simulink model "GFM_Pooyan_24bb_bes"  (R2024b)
settings: Solver=FixedStepAuto  StartTime=0.0  StopTime=1  FixedStep=Ts  RelTol=1e-3
model workspace (MAT data in the model file):
  Po = 0
  b1 = 1000.38104695
  b2 = 1006.47399607
  b3 = 1006.95432939
  b4 = 996.322108769
  b5 = 995.669039411
  b6 = 1012.96535236
  b7 = 1007.5422409
  b8 = 993.960341463
  l1 = 8282.83466164
  l10 = 5511.54621883
  l11 = 8516.9845943
  l12 = 3533.51403234
  l13 = 1255.67117866
  l14 = 1105.23671469
  l15 = 955.492069576
  l16 = 1255.83166019
  l2 = 7767.51754481
  l3 = 6680.69860842
  l4 = 3013.93364227
  l5 = 912.604633733
  l6 = 706.803488619
  l7 = 1117.39027011
  l8 = 1674.30810947
  l9 = 1971.00014576
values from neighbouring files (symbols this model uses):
  alpha_p = 0.0005    [initialcondition_gfm_Pooyan.m]    (also in initialcondition_Pooyan.m = 0.0001)
  alpha_q = 0.0001    [initialcondition_gfm_Pooyan.m]    (also in initialcondition_Pooyan.m)
  Cf = 50e-6    (= 5e-05)    [initialcondition_gfm_Pooyan.m]    (also in initialcondition_Pooyan.m)
  I_instant_limit_peak = I_instant_limit_rms * sqrt(2)    [initialcondition_gfm_Pooyan.m]
  I_overload_limit = 1.2 * I_rated_rms    [initialcondition_gfm_Pooyan.m]
  Kicc = 314.159    [initialcondition_gfm_Pooyan.m]    (also in initialcondition_Pooyan.m)
  Kivc = 400    [initialcondition_gfm_Pooyan.m]    (also in initialcondition_Pooyan.m)
  Kpcc = 31.4159    [initialcondition_gfm_Pooyan.m]    (also in initialcondition_Pooyan.m)
  Kpvc = 0.5    [initialcondition_gfm_Pooyan.m]    (also in initialcondition_Pooyan.m)
  Lf = 10e-3    (= 0.01)    [initialcondition_gfm_Pooyan.m]    (also in initialcondition_Pooyan.m)
  Lg = X_BY_R*Rg/(wn)    [initialcondition_gfm_Pooyan.m]    (also in DER_param.m = (X_BY_R_gfl * Rg) / wn_gfl; initialcondition_Pooyan.m)
  Pn = 20000    [initialcondition_gfm_Pooyan.m]    (also in initialcondition_Pooyan.m)
  Qn = 0    [initialcondition_gfm_Pooyan.m]    (also in initialcondition_Pooyan.m)
  R = (3*Vg^2)/(2*Pn)    (= 8.000067)    [initialcondition_gfm_Pooyan.m]    (also in MC2.m = (8760*SS-sum(Tdown))/(8760*SS); initialcondition_Pooyan.m)
  R_extra = (3*Vg^2)/(2*P_extra)    (= 10.666756)    [initialcondition_gfm_Pooyan.m]
  Rf = 0.1    [initialcondition_gfm_Pooyan.m]    (also in initialcondition_Pooyan.m)
  Rg = (3*Vg^2)/(2*SCR*sqrt(1+X_BY_R^2)*Pn)    [initialcondition_gfm_Pooyan.m]    (also in DER_param.m = (3 * Vg_gfl^2) / (2 * SCR_gfl * sqrt(1 + X_BY_R_gfl^2) * Pn_; initialcondition_Pooyan.m)
  tau_p = 0.031415    [initialcondition_gfm_Pooyan.m]    (also in initialcondition_Pooyan.m)
  tau_q = 0.031415    [initialcondition_gfm_Pooyan.m]    (also in initialcondition_Pooyan.m)
  Ts = 50e-6    (= 5e-05)    [initialcondition_gfm_Pooyan.m]    (also in initialcondition_Pooyan.m)
  Vdc = 700    [initialcondition_gfm_Pooyan.m]    (also in initialcondition_Pooyan.m)
  Vg = 326.6    [initialcondition_gfm_Pooyan.m]    (also in initialcondition_Pooyan.m)
  wn = 2*pi*50    (= 314.159265359)    [initialcondition_gfm_Pooyan.m]    (also in initialcondition_Pooyan.m)
undefined symbols (not defined in the file or in its folder): Ion, Lithium
libraries: simulink x6, slpidlib x5, spsThreePhaseBreakerLib x3, spsabctodq0Lib x3, spsGroundLib x3, spsThreePhaseSeriesRLCBranchLib x3, spsThreePhaseVIMeasurementLib x3, spsIGBTDiodeLib x2, spsSeriesRLCBranchLib x2, spsThreePhaseParallelRLCBranchLib x2, spsThreePhaseSourceLib x1, spsBatteryLib x1
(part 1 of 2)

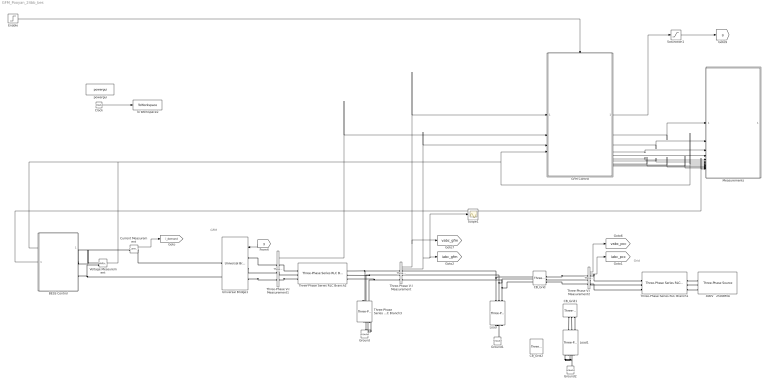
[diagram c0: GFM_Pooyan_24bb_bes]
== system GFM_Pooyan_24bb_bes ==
  note: Grid
  note: GFM
  400V   2500MVA : spsThreePhaseSourceLib/Three-Phase Source  InternalConnection=Yg  VoltagePhases=off  Voltage=Vg*sqrt(3/2)  PhaseAngle=0  Voltage_phases=[25e3 25e3 25e3]/sqrt(3)  PhaseAngles_phases=[0 -120 +120]  Frequency=50  NonIdealSource=on  SpecifyImpedance=off  Resistance=0  Inductance=0  ShortCircuitLevel=2500e6  BaseVoltage=Vg*sqrt(3/2)  XRratio=7  BusType=swing  Pref=0  Qref=0  Prefabc=[10e3, 10e3, 10e3]  Qrefabc=[0, 0, 0]  Qmin=-inf  Qmax=inf
  BESS Control : Subsystem
  CB_Grid : spsThreePhaseBreakerLib/Three-Phase Breaker  InitialState=open  SwitchA=on  SwitchB=on  SwitchC=on  SwitchTimes=[0.5]  External=off  BreakerResistance=0.01  SnubberResistance=1e6  SnubberCapacitance=inf  Measurements=None
  CB_Grid1 : spsThreePhaseBreakerLib/Three-Phase Breaker  Commented=on  InitialState=open  SwitchA=on  SwitchB=on  SwitchC=on  SwitchTimes=[1.5]  External=off  BreakerResistance=0.01  SnubberResistance=1e6  SnubberCapacitance=inf  Measurements=None
  CB_Grid2 : spsThreePhaseBreakerLib/Three-Phase Breaker  Commented=on  InitialState=closed  SwitchA=on  SwitchB=on  SwitchC=on  SwitchTimes=[1]  External=on  BreakerResistance=0.01  SnubberResistance=1e6  SnubberCapacitance=inf  Measurements=None
  Clock : Clock
  Current Measurement : spsCurrentMeasurementLib/Current Measurement  PhasorSimulation=off  OutputType=Complex  PSBequivalent=0
  Enable : Step  Time=0  SampleTime=0
  GFM Control : Subsystem
  Ground : spsGroundLib/Ground  LConnTagsString=a
  Ground1 : spsGroundLib/Ground  LConnTagsString=a
  Ground2 : spsGroundLib/Ground  Commented=on  LConnTagsString=a
  Load : spsThreePhaseParallelRLCBranchLib/Three-Phase Parallel RLC Branch  LConnTagsString=A|B|C  RConnTagsString=A|B|C  BranchType=R  Resistance=R  Inductance=1e-3  Capacitance=1e-6  Measurements=None
  Load1 : spsThreePhaseParallelRLCBranchLib/Three-Phase Parallel RLC Branch  Commented=on  LConnTagsString=A|B|C  RConnTagsString=A|B|C  BranchType=R  Resistance=R_extra  Inductance=1e-3  Capacitance=1e-6  Measurements=None
  Measurements : Subsystem
  Saturation1 : Saturate  UpperLimit=1  LowerLimit=-1
  Scope1 : Scope
  Three-Phase Series RLC Branch1 : spsThreePhaseSeriesRLCBranchLib/Three-Phase Series RLC Branch  LConnTagsString=A|B|C  RConnTagsString=A|B|C  BranchType=RL  Resistance=Rg  Inductance=Lg  Capacitance=1e-6  Measurements=None
  Three-Phase Series RLC Branch2 : spsThreePhaseSeriesRLCBranchLib/Three-Phase Series RLC Branch  LConnTagsString=A|B|C  RConnTagsString=A|B|C  BranchType=RL  Resistance=Rf  Inductance=Lf  Capacitance=1e-6  Measurements=None
  Three-Phase Series RLC Branch3 : spsThreePhaseSeriesRLCBranchLib/Three-Phase Series RLC Branch  LConnTagsString=A|B|C  RConnTagsString=A|B|C  BranchType=C  Resistance=0.1  Inductance=280e-3  Capacitance=Cf  Measurements=None
  Three-Phase V-I Measurement : spsThreePhaseVIMeasurementLib/Three-Phase V-I Measurement  VoltageMeasurement=phase-to-ground  SetLabelV=off  LabelV=Vabc  Vpu=off  VpuLL=off  CurrentMeasurement=yes  SetLabelI=off  LabelI=Iabc  Ipu=off  Pbase=100e6  Vbase=500e3  OutputType=Complex  PhasorSimulation=off  PSBequivalent=0
  Three-Phase V-I Measurement1 : spsThreePhaseVIMeasurementLib/Three-Phase V-I Measurement  VoltageMeasurement=no  SetLabelV=off  LabelV=Vabc  Vpu=off  VpuLL=off  CurrentMeasurement=yes  SetLabelI=off  LabelI=Iabc  Ipu=off  Pbase=100e6  Vbase=500e3  OutputType=Complex  PhasorSimulation=off  PSBequivalent=0
  Three-Phase V-I Measurement2 : spsThreePhaseVIMeasurementLib/Three-Phase V-I Measurement  VoltageMeasurement=phase-to-ground  SetLabelV=off  LabelV=Vabc  Vpu=off  VpuLL=off  CurrentMeasurement=yes  SetLabelI=off  LabelI=Iabc  Ipu=off  Pbase=100e6  Vbase=500e3  OutputType=Complex  PhasorSimulation=off  PSBequivalent=0
  To Workspace2 : ToWorkspace  VariableName=t  SampleTime=-1
  Universal Bridge1 : spsUniversalBridgeLib/Universal Bridge  Arms=3  SnubberResistance=1e5  SnubberCapacitance=inf  Device=Average-model based VSC  Ron=1e-3  Lon=0  ForwardVoltages="[  0  0  ]"  ForwardVoltage=0  GTOparameters=[ 10e-6 , 20e-6 ]  IGBTparameters=[ 1e-6 , 2e-6 ]  Measurements=None  Measurements_2=None  converterType=Rectifier
  Voltage Measurement : spsVoltageMeasurementLib/Voltage Measurement  PhasorSimulation=off  OutputType=Complex  PSBequivalent=0
  powergui : spspowerguiLib/powergui  Priority=1  SimulationMode=Discrete  SampleTime=Ts  frequency=50  Iterations=50  frequencyindice=0  Pbase=100e6  ErrMax=1e-4  UnitsV=kV  UnitsW=MW  buscounter=0  FunctionMessages=off  echomessages=off  EnableUseOfTLC=off  CurrentSourceSwitches=off  DisableSnubberDevices=off  DisableRonSwitches=off  DisableVfSwitches=off  DisplayEquations=off  AutomaticDiscreteSolvers=off  SolverType=Tustin  Interpol=off  ExternalGateDelay=off  methode=off  Ts=0  x0status=blocks  SPID=off  SwTol=0  HookPort=off  NonlinearTolerance=0  nMaxIteration=15  ContinueOnMaxIteration=off  RestoreLinks=warning  ResistiveCurrentMeasurement=off  Frange=[0:2:500]  Ylog=off  Xlog=on  ShowGrid=off  save=off  variable=ZData  structure=0  ZoomFFT=on  StartTime=0.0  cycles=1  DisplayStyle=1  fundamental=60  FreqAxis=off  MaxFrequency=1000  frequencyindicesteady=1  RmsSteady=1  display=off
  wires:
  [g] -> Universal Bridge1/1
  Clock/1 -> To Workspace2/1
  Three-Phase V-I Measurement2/1 -> [vabc_pcc]
  Current Measurement/1 -> [i_demand]
  Three-Phase V-I Measurement/1 -> [vabc_gfm], GFM Control/1(v_abc_gfm)
  Three-Phase V-I Measurement/2 -> Scope1/1, [iabc_gfm], GFM Control/3(i_abc_gfm)
  Three-Phase V-I Measurement1/1 -> GFM Control/2(i_abc_filter)
  Enable/1 -> GFM Control/Enable
  Voltage Measurement/1 -> Measurements/7(In7), GFM Control/4(vdc), BESS Control/1(vbus)
  GFM Control/1(g) -> Saturation1/1
  GFM Control/2(Outport) -> Measurements/1(In1)
  GFM Control/3(Outport1) -> Measurements/2(In2)
  GFM Control/4(Outport2) -> Measurements/3(In3)
  GFM Control/5(Outport3) -> Measurements/4(In4)
  GFM Control/6(Outport4) -> Measurements/5(In5)
  GFM Control/7(Outport5) -> Measurements/6(In6)
  Three-Phase V-I Measurement2/2 -> [iabc_pcc]
  GFM Control/9(CB) -> Measurements/8(CB)
  GFM Control/10(peak) -> Measurements/9(peak)
  GFM Control/11(rms) -> Measurements/10(rms)
  BESS Control/1(I_ref) -> Measurements/11(I_ref)
  Saturation1/1 -> [g]
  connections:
  Three-Phase V-I Measurement/LConn3 -- Three-Phase Series RLC Branch3/LConn3 -- Three-Phase Series RLC Branch2/RConn3
  Three-Phase V-I Measurement/LConn1 -- Three-Phase Series RLC Branch2/RConn1 -- Three-Phase Series RLC Branch3/LConn1
  Ground/LConn1 -- Three-Phase Series RLC Branch3/RConn1 -- Three-Phase Series RLC Branch3/RConn2 -- Three-Phase Series RLC Branch3/RConn3
  Three-Phase V-I Measurement1/RConn1 -- Three-Phase Series RLC Branch2/LConn1
  Three-Phase V-I Measurement1/RConn2 -- Three-Phase Series RLC Branch2/LConn2
  Three-Phase V-I Measurement/LConn2 -- Three-Phase Series RLC Branch3/LConn2 -- Three-Phase Series RLC Branch2/RConn2
  Three-Phase V-I Measurement1/RConn3 -- Three-Phase Series RLC Branch2/LConn3
  Load/LConn1 -- Three-Phase V-I Measurement/RConn1 -- CB_Grid/LConn1
  Load/LConn2 -- CB_Grid/LConn2 -- Three-Phase V-I Measurement/RConn2
  Load/LConn3 -- CB_Grid/LConn3 -- Three-Phase V-I Measurement/RConn3
  Three-Phase Series RLC Branch1/RConn1 -- 400V   2500MVA/RConn1
  Three-Phase Series RLC Branch1/RConn2 -- 400V   2500MVA/RConn2
  Three-Phase Series RLC Branch1/RConn3 -- 400V   2500MVA/RConn3
  Three-Phase V-I Measurement2/RConn1 -- Three-Phase Series RLC Branch1/LConn1
  Three-Phase V-I Measurement2/RConn2 -- Three-Phase Series RLC Branch1/LConn2
  Three-Phase V-I Measurement2/RConn3 -- Three-Phase Series RLC Branch1/LConn3
  CB_Grid/RConn1 -- Three-Phase V-I Measurement2/LConn1
  CB_Grid/RConn2 -- Three-Phase V-I Measurement2/LConn2
  CB_Grid/RConn3 -- Three-Phase V-I Measurement2/LConn3
  Load/RConn3 -- Ground1/LConn1 -- Load/RConn2 -- Load/RConn1
  Universal Bridge1/LConn1 -- Three-Phase V-I Measurement1/LConn1
  Universal Bridge1/LConn2 -- Three-Phase V-I Measurement1/LConn2
  Universal Bridge1/LConn3 -- Three-Phase V-I Measurement1/LConn3
  Voltage Measurement/LConn2 -- Universal Bridge1/RConn2 -- BESS Control/LConn2
  BESS Control/LConn1 -- Current Measurement/LConn1 -- Voltage Measurement/LConn1
  Current Measurement/RConn1 -- Universal Bridge1/RConn1
  Load1/RConn1 -- Load1/RConn3 -- Ground2/LConn1 -- Load1/RConn2
  Load1/LConn1 -- CB_Grid1/LConn1
  Load1/LConn2 -- CB_Grid1/LConn2
  Load1/LConn3 -- CB_Grid1/LConn3

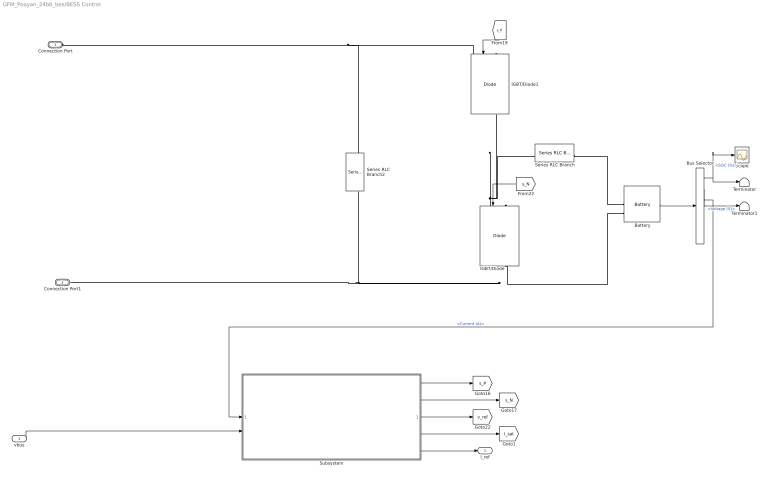
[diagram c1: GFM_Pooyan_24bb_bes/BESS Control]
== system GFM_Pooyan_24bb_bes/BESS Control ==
  vbus : Inport
  Battery : spsBatteryLib/Battery  BatType=Lithium-Ion  NomV=385  NomQ=52  SOC=90  Batt_Tr=1  PresetModel=on  MaxQ=52  MinV=288.75  FullV=448.135  Dis_rate=22.6087  R=0.074038  Normal_OP=47.0261  expZone="[415.9486      2.554783]"
  Bus Selector : BusSelector  OutputSignals=SOC (%),Voltage (V),Current (A)
  IGBT/Diode : spsIGBTDiodeLib/IGBT//Diode  Ron=1e-3  Rs=1e5  Cs=inf  Measurements=off
  IGBT/Diode1 : spsIGBTDiodeLib/IGBT//Diode  Ron=1e-3  Rs=1e5  Cs=inf  Measurements=off
  Scope : Scope
  Series RLC Branch : spsSeriesRLCBranchLib/Series RLC Branch  LConnTagsString=__new0  RConnTagsString=__new0  BranchType=RL  Resistance=0.02  Inductance=1.8e-3  SetiL0=off  InitialCurrent=0  Capacitance=1e-6  Setx0=off  InitialVoltage=0  Measurements=None
  Series RLC Branch2 : spsSeriesRLCBranchLib/Series RLC Branch  LConnTagsString=__new0  RConnTagsString=__new0  BranchType=RC  Resistance=0.05  Inductance=1e-3  SetiL0=off  InitialCurrent=0  Capacitance=470e-6  Setx0=on  InitialVoltage=385  Measurements=None
  Subsystem : Subsystem
  Terminator : Terminator
  Terminator1 : Terminator
  Connection Port : PMIOPort  Side=Left
  Connection Port1 : PMIOPort  Port=2  Side=Left
  I_ref : Outport
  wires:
  [s_N] -> IGBT/Diode/1
  Battery/1 -> Bus Selector/1
  [s_P] -> IGBT/Diode1/1
  Bus Selector/3 -> Subsystem/1(i_bat)  "<Current (A)>"
  Bus Selector/1 -> Scope/1, Terminator/1  "<SOC (%)>"
  Bus Selector/2 -> Terminator1/1  "<Voltage (V)>"
  Subsystem/1(P) -> [s_P]
  Subsystem/2(Out2) -> [s_N]
  Subsystem/3(Out3) -> [v_ref]
  vbus/1 -> Subsystem/2(Inport)
  Subsystem/4(MAX_CURRENT) -> [I_sat]
  Subsystem/5(I_ref) -> I_ref/1
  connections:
  IGBT/Diode/LConn1 -- Series RLC Branch/LConn1 -- IGBT/Diode1/RConn1
  Battery/LConn2 -- Series RLC Branch2/RConn1 -- Connection Port1/RConn1 -- IGBT/Diode/RConn1
  Connection Port/RConn1 -- Series RLC Branch2/LConn1 -- IGBT/Diode1/LConn1
  Battery/LConn1 -- Series RLC Branch/RConn1

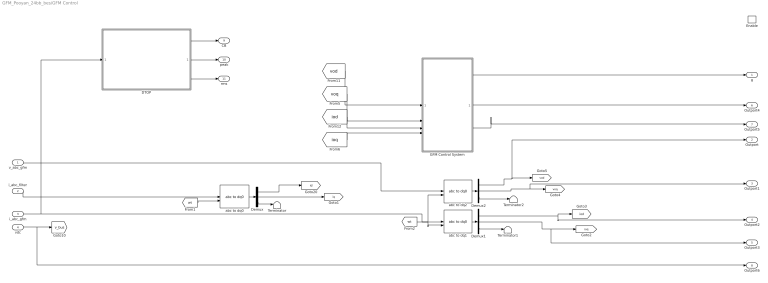
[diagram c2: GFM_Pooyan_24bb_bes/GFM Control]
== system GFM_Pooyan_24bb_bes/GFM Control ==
  v_abc_gfm : Inport
  i_abc_filter : Inport  Port=2
  i_abc_gfm : Inport  Port=3
  vdc : Inport  Port=4
  Enable : EnablePort  StatesWhenEnabling=reset
  DTOP : Subsystem
  Demux : Demux  Outputs=3
  Demux1 : Demux  Outputs=3
  Demux2 : Demux  Outputs=3
  GFM Control System : Subsystem
  Terminator : Terminator
  Terminator1 : Terminator
  Terminator2 : Terminator
  abc to dq0 : spsabctodq0Lib/abc to dq0  Alignment=90 degrees behind phase A axis
  abc to dq1 : spsabctodq0Lib/abc to dq0  Alignment=90 degrees behind phase A axis
  abc to dq2 : spsabctodq0Lib/abc to dq0  Alignment=90 degrees behind phase A axis
  g : Outport
  Outport : Outport  Port=2
  Outport1 : Outport  Port=3
  Outport2 : Outport  Port=4
  Outport3 : Outport  Port=5
  Outport4 : Outport  Port=6
  Outport5 : Outport  Port=7
  Outport6 : Outport  Port=8
  CB : Outport  Port=9
  peak : Outport  Port=10
  rms : Outport  Port=11
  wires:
  Demux1/2 -> Outport3/1, [ioq]
  [vod] -> GFM Control System/1(vod)
  Demux1/1 -> Outport2/1, [iod]
  Demux2/3 -> Terminator2/1
  Demux2/1 -> Outport/1, [vod]
  abc to dq2/1 -> Demux2/1
  Demux/1 -> [id]
  Demux/2 -> [iq]
  Demux2/2 -> Outport1/1, [voq]
  [ioq] -> GFM Control System/4(ioq)
  [wt] -> abc to dq2/2, abc to dq1/2
  i_abc_filter/1 -> abc to dq0/1
  [voq] -> GFM Control System/2(voq)
  [iod] -> GFM Control System/3(iod)
  abc to dq1/1 -> Demux1/1
  Demux/3 -> Terminator/1
  abc to dq0/1 -> Demux/1
  Demux1/3 -> Terminator1/1
  GFM Control System/1(g) -> g/1
  i_abc_gfm/1 -> DTOP/1(In), abc to dq1/1
  v_abc_gfm/1 -> abc to dq2/1
  vdc/1 -> Outport6/1, [v_bus]
  GFM Control System/3(Outport1) -> Outport5/1
  GFM Control System/2(Outport) -> Outport4/1
  [wt] -> abc to dq0/2
  DTOP/1(CB) -> CB/1
  DTOP/3(rms) -> rms/1
  DTOP/2(peak) -> peak/1

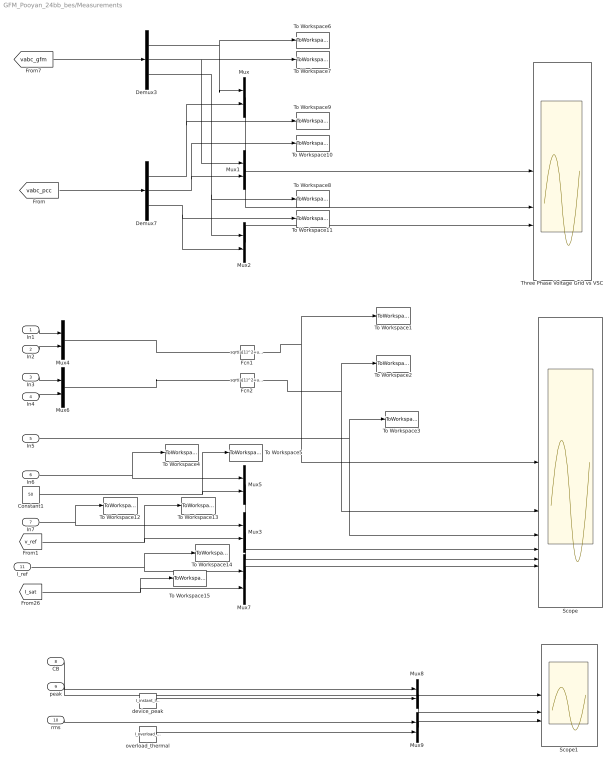
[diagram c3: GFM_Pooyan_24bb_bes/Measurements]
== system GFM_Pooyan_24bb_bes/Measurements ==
  In1 : Inport
  In2 : Inport  Port=2
  In3 : Inport  Port=3
  In4 : Inport  Port=4
  In5 : Inport  Port=5
  In6 : Inport  Port=6
  In7 : Inport  Port=7
  CB : Inport  Port=8
  peak : Inport  Port=9
  rms : Inport  Port=10
  I_ref : Inport  Port=11
  Constant1 : Constant  Value=50
  Demux3 : Demux  Outputs=3
  Demux7 : Demux  Outputs=3
  Fcn1 : Fcn  Expr=sqrt(u[1]^2+u[2]^2)
  Fcn2 : Fcn  Expr=sqrt(u[1]^2+u[2]^2)
  Mux{,1..9} (10 alike) : Mux  Inputs=2
  Scope : Scope  NumInputPorts=6
  Scope1 : Scope  NumInputPorts=3
  Three Phase Voltage Grid vs VSC : Scope  NumInputPorts=3
  To Workspace1 : ToWorkspace  VariableName=vo_GFM  SaveFormat=Timeseries  SampleTime=-1
  To Workspace10 : ToWorkspace  VariableName=Vb_grid  SaveFormat=Timeseries  SampleTime=-1
  To Workspace11 : ToWorkspace  VariableName=Vc_grid  SaveFormat=Timeseries  SampleTime=-1
  To Workspace12 : ToWorkspace  VariableName=vdc_meas_bess  SaveFormat=Timeseries  SampleTime=-1
  To Workspace13 : ToWorkspace  VariableName=vdc_set_bess  SaveFormat=Timeseries  SampleTime=-1
  To Workspace14 : ToWorkspace  VariableName=iref_bess  SaveFormat=Timeseries  SampleTime=-1
  To Workspace15 : ToWorkspace  VariableName=isat_bess  SaveFormat=Timeseries  SampleTime=-1
  To Workspace2 : ToWorkspace  VariableName=io_GFM  SaveFormat=Timeseries  SampleTime=-1
  To Workspace3 : ToWorkspace  VariableName=po_GFM1  SaveFormat=Timeseries  SampleTime=-1
  To Workspace4 : ToWorkspace  VariableName=fmeas_GFM  SaveFormat=Timeseries  SampleTime=-1
  To Workspace5 : ToWorkspace  VariableName=fset_GFM  SaveFormat=Timeseries  SampleTime=-1
  To Workspace6 : ToWorkspace  VariableName=Va_gfm  SaveFormat=Timeseries  SampleTime=-1
  To Workspace7 : ToWorkspace  VariableName=Vb_gfm  SaveFormat=Timeseries  SampleTime=-1
  To Workspace8 : ToWorkspace  VariableName=Vc_gfm  SaveFormat=Timeseries  SampleTime=-1
  To Workspace9 : ToWorkspace  VariableName=Va_grid  SaveFormat=Timeseries  SampleTime=-1
  device_peak : Constant  Value=I_instant_limit_peak
  overload_thermal : Constant  Value=I_overload_limit
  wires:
  [vabc_gfm] -> Demux3/1
  Constant1/1 -> To Workspace5/1, Mux5/2
  [vabc_pcc] -> Demux7/1
  Demux3/2 -> To Workspace7/1, Mux1/1
  In1/1 -> Mux4/1
  In2/1 -> Mux4/2
  Demux3/1 -> To Workspace6/1, Mux/1
  In3/1 -> Mux6/1
  In4/1 -> Mux6/2
  Mux4/1 -> Fcn1/1
  Demux3/3 -> Mux2/1, To Workspace8/1
  Demux7/1 -> Mux/2, To Workspace9/1
  Demux7/2 -> To Workspace10/1, Mux1/2
  [v_ref] -> To Workspace13/1, Mux3/2
  Demux7/3 -> Mux2/2, To Workspace11/1
  Mux6/1 -> Fcn2/1
  In6/1 -> To Workspace4/1, Mux5/1
  In7/1 -> To Workspace12/1, Mux3/1
  [I_sat] -> To Workspace15/1, Mux7/2
  Mux/1 -> Three Phase Voltage Grid vs VSC/1
  Mux1/1 -> Three Phase Voltage Grid vs VSC/2
  Mux2/1 -> Three Phase Voltage Grid vs VSC/3
  Fcn1/1 -> To Workspace1/1, Scope/1
  Fcn2/1 -> To Workspace2/1, Scope/2
  In5/1 -> To Workspace3/1, Scope/3
  Mux5/1 -> Scope/4
  Mux7/1 -> Scope/6
  Mux3/1 -> Scope/5
  CB/1 -> Scope1/1
  peak/1 -> Mux8/1
  device_peak/1 -> Mux8/2
  Mux8/1 -> Scope1/2
  rms/1 -> Mux9/1
  overload_thermal/1 -> Mux9/2
  Mux9/1 -> Scope1/3
  I_ref/1 -> To Workspace14/1, Mux7/1

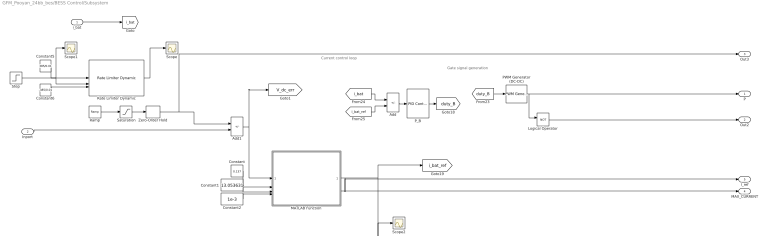
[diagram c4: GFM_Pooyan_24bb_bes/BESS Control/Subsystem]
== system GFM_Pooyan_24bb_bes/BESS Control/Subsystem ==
  note: Current control loop
  note: Gate signal generation
  i_bat : Inport
  Inport : Inport  Port=2
  Add : Sum  Inputs=+-
  Add1 : Sum  Inputs=+-
  Constant : Constant  Value=0.137
  Constant1 : Constant  Value=13.053631
  Constant2 : Constant  Value=1e-3
  Constant5 : Constant  Commented=on  Value=385/0.01
  Constant6 : Constant  Commented=on  Value=-385/0.01
  Logical Operator : Logic  Operator=NOT  AllPortsSameDT=off  OutDataTypeStr=boolean
  MATLAB Function : MATLAB Function  TreatAsAtomicUnit=on
  PWM Generator (DC-DC) : spsPWMGeneratorDCDCLib/PWM Generator (DC-DC)  Fsw=10000  Ts=1/10000
  P_B : slpidlib/PID Controller  Controller=PI  Form=Parallel  TimeDomain=Discrete-time  UseExternalTs=off  SampleTime=200e-6  IntegratorMethod=Forward Euler  FilterMethod=Forward Euler  ControllerParametersSource=internal  P=0.015756  I=0.179520  UseKiTs=off  D=0  UseExternalDerivativeSource=off  N=100  UseFilter=on  TunerSelectOption=Transfer Function Based (PID Tuner App)  InitialConditionSource=internal  InitialConditionForIntegrator=0  InitialConditionForFilter=0  DifferentiatorICPrevScaledInput=0  ExternalReset=none  TrackingMode=off  Kt=1  LimitOutput=on  SatLimitsSource=internal  UpperSaturationLimit=0.95  LowerSaturationLimit=0  LinearizeAsGain=off  AntiWindupMode=none  Kb=1  LimitIntegrator=off  UpperIntegratorSaturationLimit=inf  LowerIntegratorSaturationLimit=-inf  POutMin=[]  POutMax=[]  IOutMin=[]  IOutMax=[]  DOutMin=[]  DOutMax=[]  NOutMin=[]  NOutMax=[]  SumOutMin=[]  SumOutMax=[]  SaturationOutMin=[]  SaturationOutMax=[]  PParamMin=[]  PParamMax=[]  IParamMin=[]  IParamMax=[]  DParamMin=[]  DParamMax=[]  NParamMin=[]  NParamMax=[]  KbParamMin=[]  KbParamMax=[]  KtParamMin=[]  KtParamMax=[]  KbOutMin=[]  KbOutMax=[]  KtOutMin=[]  KtOutMax=[]  IntegratorOutMin=[]  IntegratorOutMax=[]  FilterOutMin=[]  FilterOutMax=[]  SumI1OutMin=[]  SumI1OutMax=[]  SumI2OutMin=[]  SumI2OutMax=[]  SumI3OutMin=[]  SumI3OutMax=[]  SumI4OutMin=[]  SumI4OutMax=[]  SumDOutMin=[]  SumDOutMax=[]  DifferentiatorOutMin=[]  DifferentiatorOutMax=[]  FilterDiffOutCoefMin=[]  FilterDiffOutCoefMax=[]  ReciprocalOutMin=[]  ReciprocalOutMax=[]  SumDenOutMin=[]  SumDenOutMax=[]  SumNumOutMin=[]  SumNumOutMax=[]  DivideOutMin=[]  DivideOutMax=[]  UdiffTsProdOutMin=[]  UdiffTsProdOutMax=[]  NTsProdOutMin=[]  NTsProdOutMax=[]  UintegralTsProdOutMin=[]  UintegralTsProdOutMax=[]  UngainTsProdOutMin=[]  UngainTsProdOutMax=[]  ClampingZeroOutDataTypeStr=Inherit: Inherit via back propagation  ClampingZeroOutMin=[]  ClampingZeroOutMax=[]  FilterDenConstantOutDataTypeStr=Inherit: Inherit via back propagation  FilterDenConstantOutMin=[]  FilterDenConstantOutMax=[]  PCopyOutDataTypeStr=Inherit: Inherit via back propagation  PCopyOutMin=[]  PCopyOutMax=[]  NCopyOutDataTypeStr=Inherit: Inherit via back propagation  NCopyOutMin=[]  NCopyOutMax=[]  IntegratorContinuousStateAttributes=''  IntegratorStateMustResolveToSignalObject=off  IntegratorRTWStateStorageClass=Auto  FilterContinuousStateAttributes=''  FilterStateMustResolveToSignalObject=off  FilterRTWStateStorageClass=Auto  ParallelPVariant=InternalParameters  IdealPVariant=Disabled  IVariant=InternalParameters  DVariant=Disabled  IntegratorVariant=Discrete  SatVariant=Enabled  AWVariant=Passthrough  PCopyVariant=Disabled  TRVariant=Disabled  FdbkBlocksVariant=Forward  IdealPFdbkVariant=Disabled  SatFdbkVariant=Disabled  DerivativeFilterVariant=Disabled  NVariant=Disabled  NCopyVariant=Disabled_SignalSpec  FilterICVariant=Disabled  IntegratorICVariant=InternalICs  ExternalResetVariant=Disabled  TRSumVariant=Passthrough  SumFdbkVariant=Disabled  SumVariant=Sum_PI  TsampFilterVariant=InternalTs  TsampNgainVariant=Passthrough  TsampIntegralVariant=Disabled_SignalSpec  ExternalSaturationOutDataTypeStr=Inherit: Same as second input  DerivativeSourceVariant=Disabled  PreIntVariant=InternalPreInt
  Ramp : simulink/Sources/Ramp  slope=315/0.01  start=0  InitialOutput=385
  Rate Limiter Dynamic : simulink/Discontinuities/Rate Limiter Dynamic  Commented=on
  Saturation : Saturate  UpperLimit=700  LowerLimit=-385
  Scope : Scope
  Scope1 : Scope
  Scope2 : Scope
  Step : Step  Commented=on  Time=0.01  Before=385  After=700  SampleTime=0
  Zero-Order Hold : ZeroOrderHold  SampleTime=-1
  P : Outport
  Out2 : Outport  Port=2
  Out3 : Outport  Port=3
  MAX_CURRENT : Outport  Port=4
  I_ref : Outport  Port=5
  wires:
  [duty_B] -> PWM Generator (DC-DC)/1
  [i_bat] -> Add/1
  [i_bat_ref] -> Add/2
  Constant2/1 -> MATLAB Function/4(dt)
  PWM Generator (DC-DC)/1 -> P/1, Logical Operator/1
  MATLAB Function/2(MAX_CURRENT) -> MAX_CURRENT/1
  P_B/1 -> [duty_B]
  Constant/1 -> MATLAB Function/2(Kp)
  Add/1 -> P_B/1
  Logical Operator/1 -> Out2/1
  MATLAB Function/1(control_signal) -> I_ref/1, Scope2/1, [i_bat_ref]
  Constant1/1 -> MATLAB Function/3(Ki)
  Add1/1 -> [V_dc_err], MATLAB Function/1(error)
  Inport/1 -> Add1/2
  Rate Limiter Dynamic/1 -> Scope/1
  i_bat/1 -> [i_bat]
  Constant6/1 -> Rate Limiter Dynamic/3
  Constant5/1 -> Rate Limiter Dynamic/1
  Step/1 -> Scope1/1, Rate Limiter Dynamic/2
  Ramp/1 -> Saturation/1
  Saturation/1 -> Zero-Order Hold/1
  Zero-Order Hold/1 -> Out3/1, Add1/1

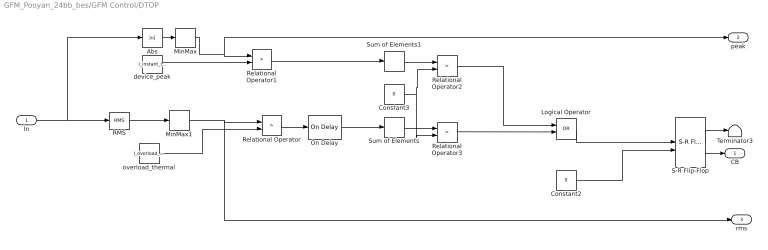
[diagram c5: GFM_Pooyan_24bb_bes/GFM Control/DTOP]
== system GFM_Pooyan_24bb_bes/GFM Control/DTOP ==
  In : Inport
  Abs : Abs
  Constant2 : Constant  Value=0  OutDataTypeStr=boolean
  Constant3 : Constant  Value=0
  Logical Operator : Logic  Operator=OR  AllPortsSameDT=off  OutDataTypeStr=boolean
  MinMax : MinMax  Function=max
  MinMax1 : MinMax  Function=max
  On Delay : spsOnDelayLib/On Delay  DelayType=On delay  delay=0.5  ic=0  Ts=0
  RMS : spsRMSLib/RMS  TrueRMS=on  Freq=50  RMSInit=120  Ts=0
  Relational Operator{,1..3} (4 alike) : RelationalOperator  Operator=>  OutDataTypeStr=boolean  RndMeth=Simplest
  S-R Flip-Flop : simulink_extras/Flip Flops/S-R Flip-Flop  initial_condition=0
  Sum of Elements : Sum  Inputs=+
  Sum of Elements1 : Sum  Inputs=+
  Terminator3 : Terminator
  device_peak : Constant  Value=I_instant_limit_peak
  overload_thermal : Constant  Value=I_overload_limit
  CB : Outport
  peak : Outport  Port=2
  rms : Outport  Port=3
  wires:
  Relational Operator1/1 -> Sum of Elements1/1
  device_peak/1 -> Relational Operator1/2
  Logical Operator/1 -> S-R Flip-Flop/1
  overload_thermal/1 -> Relational Operator/2
  Constant2/1 -> S-R Flip-Flop/2
  On Delay/1 -> Sum of Elements/1
  Relational Operator/1 -> On Delay/1
  In/1 -> Abs/1, RMS/1
  Sum of Elements1/1 -> Relational Operator2/1
  Constant3/1 -> Relational Operator2/2, Relational Operator3/2
  Sum of Elements/1 -> Relational Operator3/1
  Relational Operator3/1 -> Logical Operator/2
  Relational Operator2/1 -> Logical Operator/1
  Abs/1 -> MinMax/1
  MinMax/1 -> peak/1, Relational Operator1/1
  RMS/1 -> MinMax1/1
  MinMax1/1 -> rms/1, Relational Operator/1
  S-R Flip-Flop/1 -> Terminator3/1
  S-R Flip-Flop/2 -> CB/1

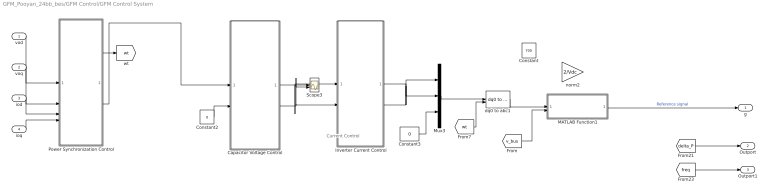
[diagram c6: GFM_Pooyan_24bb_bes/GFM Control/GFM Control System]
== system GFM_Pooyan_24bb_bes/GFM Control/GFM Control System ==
  note: Current Control
  vod : Inport
  voq : Inport  Port=2
  iod : Inport  Port=3
  ioq : Inport  Port=4
  Capacitor Voltage Control : Subsystem
  Constant : Constant  Value=700
  Constant2 : Constant  Value=0
  Constant3 : Constant  Value=0
  Inverter Current Control : Subsystem
  MATLAB Function1 : MATLAB Function  TreatAsAtomicUnit=on
  Mux3 : Mux  Inputs=3
  Power Synchronization Control : Subsystem
  Scope3 : Scope  NumInputPorts=2
  dq0 to abc1 : spsdq0toabcLib/dq0 to abc  Alignment=90 degrees behind phase A axis
  norm2 : Gain  Gain=2/Vdc
  g : Outport
  Outport : Outport  Port=2
  Outport1 : Outport  Port=3
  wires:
  Inverter Current Control/2(vqt) -> Mux3/2
  voq/1 -> Power Synchronization Control/2(voq)
  Constant2/1 -> Capacitor Voltage Control/2(voqref)
  Constant3/1 -> Mux3/3
  ioq/1 -> Power Synchronization Control/4(ioq)
  Capacitor Voltage Control/1(idref) -> Scope3/1, Inverter Current Control/1(idref)
  Power Synchronization Control/2(vdref) -> Capacitor Voltage Control/1(vodref)
  Inverter Current Control/1(vdt) -> Mux3/1
  Mux3/1 -> dq0 to abc1/1
  vod/1 -> Power Synchronization Control/1(vod)
  iod/1 -> Power Synchronization Control/3(iod)
  [wt] -> dq0 to abc1/2
  Capacitor Voltage Control/2(iqref) -> Scope3/2, Inverter Current Control/2(iqref)
  Power Synchronization Control/1(wt) -> [wt]
  [delta_P] -> Outport/1
  [freq] -> Outport1/1
  [v_bus] -> MATLAB Function1/2(Vdc_filtered)
  dq0 to abc1/1 -> MATLAB Function1/1(u)
  MATLAB Function1/1(y) -> g/1  "Reference signal"

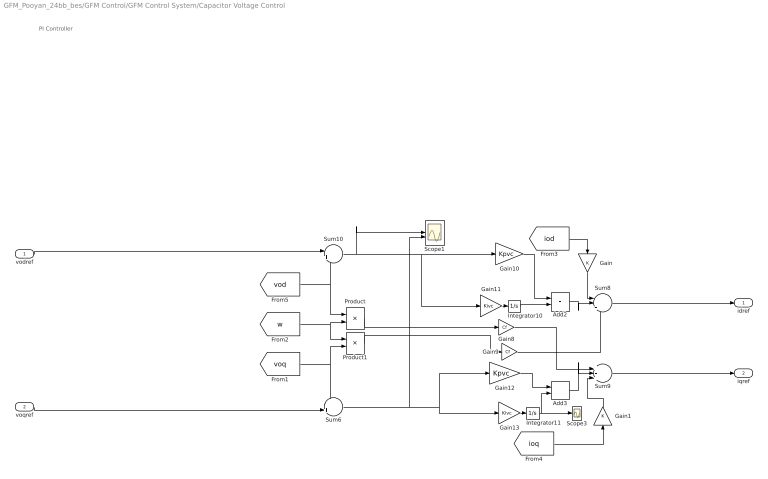
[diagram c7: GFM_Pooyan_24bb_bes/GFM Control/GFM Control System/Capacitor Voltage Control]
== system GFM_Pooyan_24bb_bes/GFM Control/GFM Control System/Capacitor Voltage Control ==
  note: PI Controller
  vodref : Inport
  voqref : Inport  Port=2
  Add2 : Sum
  Add3 : Sum
  Gain : Gain
  Gain1 : Gain
  Gain10 : Gain  Gain=Kpvc
  Gain11 : Gain  Gain=Kivc
  Gain12 : Gain  Gain=Kpvc
  Gain13 : Gain  Gain=Kivc
  Gain8 : Gain  Gain=Cf
  Gain9 : Gain  Gain=Cf
  Integrator10 : Integrator
  Integrator11 : Integrator
  Product : Product
  Product1 : Product
  Scope1 : Scope  NumInputPorts=2
  Scope3 : Scope
  Sum10 : Sum  Inputs=|+-
  Sum6 : Sum  Inputs=-+|
  Sum8 : Sum  Inputs=|++-
  Sum9 : Sum  Inputs=+++|
  idref : Outport
  iqref : Outport  Port=2
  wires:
  Gain12/1 -> Add3/1
  voqref/1 -> Sum6/2
  Gain13/1 -> Integrator11/1
  Gain8/1 -> Sum9/1
  [vod] -> Product/1, Sum10/2
  [voq] -> Product1/2, Sum6/1
  Integrator11/1 -> Add3/2, Scope3/1
  Gain11/1 -> Integrator10/1
  Gain10/1 -> Add2/1
  Add3/1 -> Sum9/2
  Integrator10/1 -> Add2/2
  vodref/1 -> Sum10/1
  [w] -> Product1/1, Product/2
  Product/1 -> Gain8/1
  Product1/1 -> Gain9/1
  Sum8/1 -> idref/1
  Sum9/1 -> iqref/1
  Add2/1 -> Sum8/2
  Gain9/1 -> Sum8/3
  [iod] -> Gain/1
  Gain/1 -> Sum8/1
  [ioq] -> Gain1/1
  Gain1/1 -> Sum9/3
  Sum10/1 -> Gain11/1, Gain10/1, Scope1/1
  Sum6/1 -> Gain13/1, Gain12/1, Scope1/2

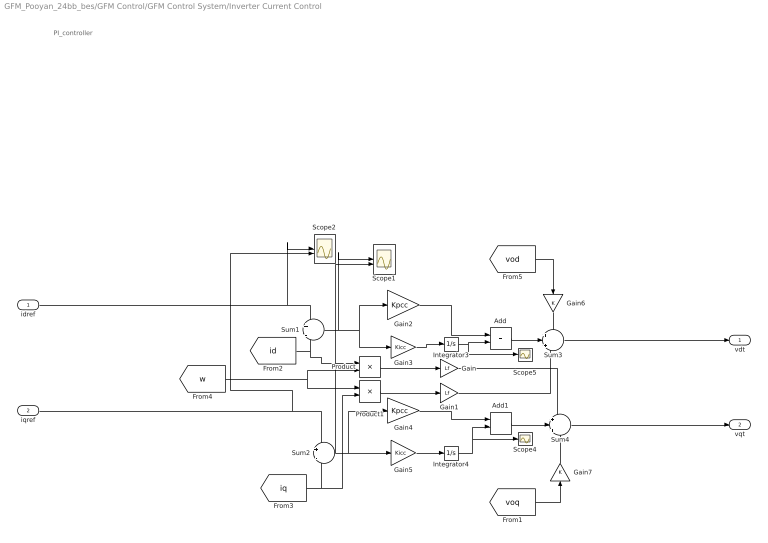
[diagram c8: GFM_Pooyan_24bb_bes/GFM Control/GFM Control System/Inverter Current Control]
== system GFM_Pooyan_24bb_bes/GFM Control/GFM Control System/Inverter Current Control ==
  note: PI_controller
  idref : Inport
  iqref : Inport  Port=2
  Add : Sum
  Add1 : Sum
  Gain : Gain  Gain=Lf
  Gain1 : Gain  Gain=Lf
  Gain2 : Gain  Gain=Kpcc
  Gain3 : Gain  Gain=Kicc
  Gain4 : Gain  Gain=Kpcc
  Gain5 : Gain  Gain=Kicc
  Gain6 : Gain
  Gain7 : Gain
  Integrator3 : Integrator
  Integrator4 : Integrator
  Product : Product
  Product1 : Product
  Scope1 : Scope  NumInputPorts=2
  Scope2 : Scope  NumInputPorts=2
  Scope4 : Scope
  Scope5 : Scope
  Sum1 : Sum  Inputs=+|-
  Sum2 : Sum  Inputs=+|-
  Sum3 : Sum  Inputs=+|+|-
  Sum4 : Sum  Inputs=+|+|+
  vdt : Outport
  vqt : Outport  Port=2
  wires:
  Gain3/1 -> Integrator3/1
  Integrator4/1 -> Scope4/1, Add1/2
  Add/1 -> Sum3/2
  Gain4/1 -> Add1/1
  Add1/1 -> Sum4/2
  Gain2/1 -> Add/1
  Gain/1 -> Sum4/1
  Gain1/1 -> Sum3/3
  Integrator3/1 -> Scope5/1, Add/2
  Gain5/1 -> Integrator4/1
  iqref/1 -> Scope2/2, Sum2/1
  [iq] -> Product1/2, Sum2/2
  idref/1 -> Scope2/1, Sum1/1
  [id] -> Product/1, Sum1/2
  Product/1 -> Gain/1
  Product1/1 -> Gain1/1
  [w] -> Product1/1, Product/2
  [vod] -> Gain6/1
  [voq] -> Gain7/1
  Gain6/1 -> Sum3/1
  Gain7/1 -> Sum4/3
  Sum3/1 -> vdt/1
  Sum4/1 -> vqt/1
  Sum1/1 -> Scope1/1, Gain2/1, Gain3/1
  Sum2/1 -> Scope1/2, Gain5/1, Gain4/1

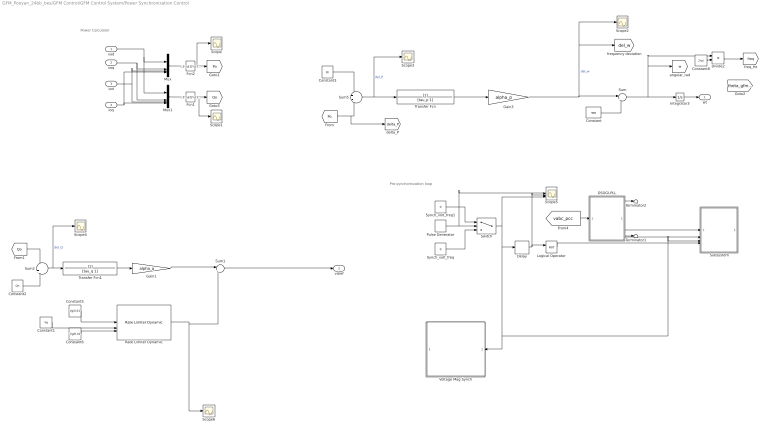
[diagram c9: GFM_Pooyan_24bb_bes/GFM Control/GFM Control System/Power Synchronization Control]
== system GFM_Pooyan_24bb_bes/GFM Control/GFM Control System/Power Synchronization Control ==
  note: Pre-synchornization loop
  note: Power Calculator
  vod : Inport
  voq : Inport  Port=2
  iod : Inport  Port=3
  ioq : Inport  Port=4
  Constant : Constant  Value=wn
  Constant1 : Constant  Value=Vg
  Constant2 : Constant  Value=Qn
  Constant3 : Constant  Value=Pn
  Constant5 : Constant  Value=Vg/0.01
  Constant6 : Constant  Value=-Vg/0.01
  Constant8 : Constant  Value=2*pi
  DSOGI-PLL : Subsystem  Commented=on
  Delay : Delay  Commented=on  DelayLength=1
  Divide2 : Product  Inputs=*/
  Fcn1 : Fcn  Expr=1.5*(u[2]*u[3]-u[1]*u[4])
  Fcn2 : Fcn  Expr=1.5*(u[1]*u[3]+u[2]*u[4])
  Gain1 : Gain  Gain=alpha_q
  Gain3 : Gain  Gain=alpha_p
  Integrator3 : Integrator
  Logical Operator : Logic  Commented=on  Operator=NOT  AllPortsSameDT=off  OutDataTypeStr=boolean
  Mux : Mux
  Mux1 : Mux
  Pulse Generator : DiscretePulseGenerator  Commented=on  PulseType=Time based  Period=10  PulseWidth=50  PhaseDelay=3
  Rate Limiter Dynamic : simulink/Discontinuities/Rate Limiter Dynamic
  Scope{,1..4,6} (6 alike) : Scope
  Scope5 : Scope  NumInputPorts=3
  Subsystem : Subsystem  Commented=on
  Sum : Sum  Inputs=|++
  Sum1 : Sum  Inputs=|++
  Sum2 : Sum  Inputs=-+
  Sum5 : Sum  Inputs=+-
  Switch : Switch  Commented=on  Criteria=u2 > Threshold
  Synch_volt_freq : Constant  Commented=on  Value=0
  Synch_volt_freq1 : Constant  Commented=on  Value=0
  Terminator1 : Terminator
  Terminator2 : Terminator
  Transfer Fcn : TransferFcn  Denominator=[tau_p 1]  ParameterTunability=Unconstrained
  Transfer Fcn1 : TransferFcn  Denominator=[tau_q 1]  ParameterTunability=Unconstrained
  Voltage Mag Synch : Subsystem  Commented=on
  wt : Outport
  vdref : Outport  Port=2
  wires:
  ioq/1 -> Mux/4, Mux1/4
  iod/1 -> Mux/3, Mux1/3
  voq/1 -> Mux1/2, Mux/2
  Gain1/1 -> Sum1/1
  Mux1/1 -> Fcn1/1
  Mux/1 -> Fcn2/1
  Integrator3/1 -> wt/1
  vod/1 -> Mux1/1, Mux/1
  Sum2/1 -> Scope4/1, Transfer Fcn1/1  "del_Q"
  Fcn2/1 -> Scope/1, [Po]
  Fcn1/1 -> Scope1/1, [Qo]
  [Qo] -> Sum2/1
  Transfer Fcn/1 -> Gain3/1
  Sum5/1 -> Scope3/1, Transfer Fcn/1  "del_P"
  Transfer Fcn1/1 -> Gain1/1
  Gain3/1 -> Scope2/1, [del_w], Sum/1  "del_w"
  Constant2/1 -> Sum2/2
  [Po] -> [delta_P], Sum5/2
  Sum1/1 -> vdref/1
  DSOGI-PLL/1(Valp_bet+) -> Terminator2/1
  DSOGI-PLL/2(w_pcc) -> Subsystem/1(w_pcc)
  [vabc_pcc] -> DSOGI-PLL/1(abc)
  DSOGI-PLL/4(f) -> Terminator1/1
  DSOGI-PLL/3(theta_pcc) -> Subsystem/2(theta_pcc)
  Logical Operator/1 -> Subsystem/4(connect)
  Synch_volt_freq1/1 -> Switch/1
  Pulse Generator/1 -> Scope5/1, Switch/2
  Synch_volt_freq/1 -> Switch/3
  Switch/1 -> Subsystem/3(sync), Voltage Mag Synch/1(u), Delay/1, Scope5/3
  Constant8/1 -> Divide2/2
  Delay/1 -> Scope5/2, Logical Operator/1
  Divide2/1 -> [freq]
  Constant3/1 -> Sum5/1
  Constant/1 -> Sum/2
  Sum/1 -> Divide2/1, [w], Integrator3/1
  Constant1/1 -> Rate Limiter Dynamic/2
  Constant6/1 -> Rate Limiter Dynamic/3
  Constant5/1 -> Rate Limiter Dynamic/1
  Rate Limiter Dynamic/1 -> Sum1/2, Scope6/1

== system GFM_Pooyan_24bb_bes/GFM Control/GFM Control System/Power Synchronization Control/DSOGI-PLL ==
  abc : Inport
  1 : Constant  Value=0
  Demux2 : Demux  Outputs=2
  K : Gain  Gain=0.5
  K1 : Gain  Gain=0.5
  Mux15 : Mux  Inputs=2
  Mux2 : Mux  Inputs=2
  SOGI-QSG1 : Subsystem
  SOGI-QSG2 : Subsystem
  SRF-PLL : Subsystem
  Sum1 : Sum  Inputs=|+-
  Sum2 : Sum  Inputs=|++
  abc to alpha-beta : Subsystem
  hr : Gain
  Valp_bet+ : Outport  VectorParamsAs1DForOutWhenUnconnected=off
  w_pcc : Outport  Port=2  VectorParamsAs1DForOutWhenUnconnected=off
  theta_pcc : Outport  Port=3  VectorParamsAs1DForOutWhenUnconnected=off
  f : Outport  Port=4  VectorParamsAs1DForOutWhenUnconnected=off
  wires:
  abc/1 -> abc to alpha-beta/1(abc)
  SOGI-QSG1/1(vad) -> Sum1/1
  Demux2/1 -> SOGI-QSG1/1(Va)
  abc to alpha-beta/1(al_be) -> Demux2/1
  Demux2/2 -> SOGI-QSG2/2(Vb)
  SOGI-QSG2/1(vbd) -> Sum2/2
  SOGI-QSG2/2(vbq) -> Sum1/2
  Sum1/1 -> K/1
  K/1 -> Mux2/1
  SOGI-QSG1/2(vaq) -> Sum2/1
  Sum2/1 -> K1/1
  K1/1 -> Mux2/2
  SRF-PLL/1(theta_pcc) -> theta_pcc/1
  SRF-PLL/2(f) -> hr/1, f/1
  Mux15/1 -> SRF-PLL/1(al-be-0)
  1/1 -> Mux15/2
  Mux2/1 -> Valp_bet+/1, Mux15/1
  hr/1 -> SOGI-QSG1/2(f), SOGI-QSG2/1(f)
  SRF-PLL/3(w_pcc) -> w_pcc/1

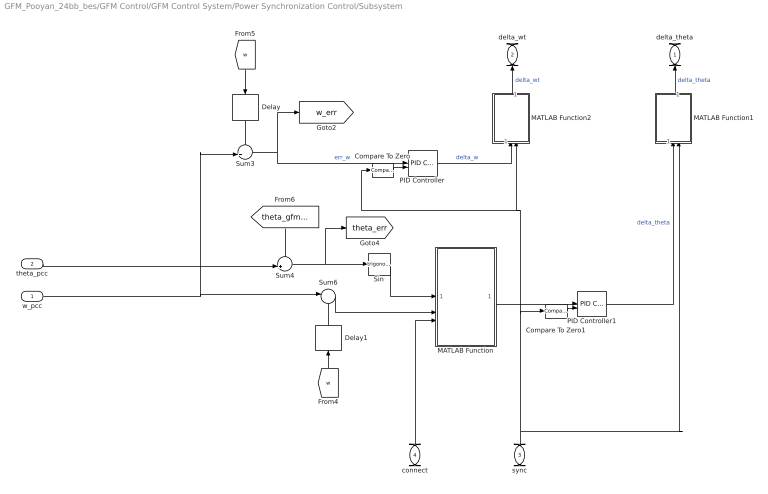
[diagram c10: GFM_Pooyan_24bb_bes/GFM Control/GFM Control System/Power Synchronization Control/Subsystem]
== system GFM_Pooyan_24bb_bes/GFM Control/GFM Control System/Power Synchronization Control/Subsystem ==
  w_pcc : Inport
  theta_pcc : Inport  Port=2
  sync : Inport  Port=3
  connect : Inport  Port=4
  Compare To Zero : simulink/Logic and Bit Operations/Compare To Zero  relop===  OutDataTypeStr=boolean
  Compare To Zero1 : simulink/Logic and Bit Operations/Compare To Zero  relop===  OutDataTypeStr=boolean
  Delay : Delay  DelayLength=1  InputProcessing=Columns as channels (frame based)
  Delay1 : Delay  DelayLength=1  InputProcessing=Columns as channels (frame based)
  MATLAB Function : MATLAB Function  TreatAsAtomicUnit=on
  MATLAB Function1 : MATLAB Function  TreatAsAtomicUnit=on
  MATLAB Function2 : MATLAB Function  TreatAsAtomicUnit=on
  PID Controller : slpidlib/PID Controller  Controller=PI  Form=Parallel  TimeDomain=Discrete-time  UseExternalTs=off  SampleTime=-1  IntegratorMethod=Forward Euler  FilterMethod=Forward Euler  ControllerParametersSource=internal  P=0.2  I=40  UseKiTs=off  D=0  UseExternalDerivativeSource=off  N=100  UseFilter=on  TunerSelectOption=Transfer Function Based (PID Tuner App)  InitialConditionSource=internal  InitialConditionForIntegrator=0  InitialConditionForFilter=0  DifferentiatorICPrevScaledInput=0  ExternalReset=level  TrackingMode=off  Kt=1  LimitOutput=off  SatLimitsSource=internal  UpperSaturationLimit=inf  LowerSaturationLimit=-inf  LinearizeAsGain=on  AntiWindupMode=none  Kb=1  LimitIntegrator=off  UpperIntegratorSaturationLimit=inf  LowerIntegratorSaturationLimit=-inf  POutMin=[]  POutMax=[]  IOutMin=[]  IOutMax=[]  DOutMin=[]  DOutMax=[]  NOutMin=[]  NOutMax=[]  SumOutMin=[]  SumOutMax=[]  SaturationOutMin=[]  SaturationOutMax=[]  PParamMin=[]  PParamMax=[]  IParamMin=[]  IParamMax=[]  DParamMin=[]  DParamMax=[]  NParamMin=[]  NParamMax=[]  KbParamMin=[]  KbParamMax=[]  KtParamMin=[]  KtParamMax=[]  KbOutMin=[]  KbOutMax=[]  KtOutMin=[]  KtOutMax=[]  IntegratorOutMin=[]  IntegratorOutMax=[]  FilterOutMin=[]  FilterOutMax=[]  SumI1OutMin=[]  SumI1OutMax=[]  SumI2OutMin=[]  SumI2OutMax=[]  SumI3OutMin=[]  SumI3OutMax=[]  SumI4OutMin=[]  SumI4OutMax=[]  SumDOutMin=[]  SumDOutMax=[]  DifferentiatorOutMin=[]  DifferentiatorOutMax=[]  FilterDiffOutCoefMin=[]  FilterDiffOutCoefMax=[]  ReciprocalOutMin=[]  ReciprocalOutMax=[]  SumDenOutMin=[]  SumDenOutMax=[]  SumNumOutMin=[]  SumNumOutMax=[]  DivideOutMin=[]  DivideOutMax=[]  UdiffTsProdOutMin=[]  UdiffTsProdOutMax=[]  NTsProdOutMin=[]  NTsProdOutMax=[]  UintegralTsProdOutMin=[]  UintegralTsProdOutMax=[]  UngainTsProdOutMin=[]  UngainTsProdOutMax=[]  ClampingZeroOutDataTypeStr=Inherit: Inherit via back propagation  ClampingZeroOutMin=[]  ClampingZeroOutMax=[]  FilterDenConstantOutDataTypeStr=Inherit: Inherit via back propagation  FilterDenConstantOutMin=[]  FilterDenConstantOutMax=[]  PCopyOutDataTypeStr=Inherit: Inherit via back propagation  PCopyOutMin=[]  PCopyOutMax=[]  NCopyOutDataTypeStr=Inherit: Inherit via back propagation  NCopyOutMin=[]  NCopyOutMax=[]  IntegratorContinuousStateAttributes=''  IntegratorStateMustResolveToSignalObject=off  IntegratorRTWStateStorageClass=Auto  FilterContinuousStateAttributes=''  FilterStateMustResolveToSignalObject=off  FilterRTWStateStorageClass=Auto  ParallelPVariant=InternalParameters  IdealPVariant=Disabled  IVariant=InternalParameters  DVariant=Disabled  IntegratorVariant=Discrete  SatVariant=Disabled  AWVariant=Passthrough  PCopyVariant=Disabled  TRVariant=Disabled  FdbkBlocksVariant=Forward  IdealPFdbkVariant=Disabled  SatFdbkVariant=Disabled  DerivativeFilterVariant=Disabled  NVariant=Disabled  NCopyVariant=Disabled_SignalSpec  FilterICVariant=Disabled  IntegratorICVariant=InternalICs  ExternalResetVariant=ExternalReset  TRSumVariant=Passthrough  SumFdbkVariant=Disabled  SumVariant=Sum_PI  TsampFilterVariant=InternalTs  TsampNgainVariant=Passthrough  TsampIntegralVariant=Disabled_SignalSpec  ExternalSaturationOutDataTypeStr=Inherit: Same as second input  DerivativeSourceVariant=Disabled  PreIntVariant=InternalPreInt
  PID Controller1 : slpidlib/PID Controller  Controller=PI  Form=Parallel  TimeDomain=Discrete-time  UseExternalTs=off  SampleTime=-1  IntegratorMethod=Forward Euler  FilterMethod=Forward Euler  ControllerParametersSource=internal  P=1  I=30  UseKiTs=off  D=0  UseExternalDerivativeSource=off  N=100  UseFilter=on  TunerSelectOption=Transfer Function Based (PID Tuner App)  InitialConditionSource=internal  InitialConditionForIntegrator=0  InitialConditionForFilter=0  DifferentiatorICPrevScaledInput=0  ExternalReset=level  TrackingMode=off  Kt=1  LimitOutput=off  SatLimitsSource=internal  UpperSaturationLimit=inf  LowerSaturationLimit=-inf  LinearizeAsGain=on  AntiWindupMode=none  Kb=1  LimitIntegrator=off  UpperIntegratorSaturationLimit=inf  LowerIntegratorSaturationLimit=-inf  POutMin=[]  POutMax=[]  IOutMin=[]  IOutMax=[]  DOutMin=[]  DOutMax=[]  NOutMin=[]  NOutMax=[]  SumOutMin=[]  SumOutMax=[]  SaturationOutMin=[]  SaturationOutMax=[]  PParamMin=[]  PParamMax=[]  IParamMin=[]  IParamMax=[]  DParamMin=[]  DParamMax=[]  NParamMin=[]  NParamMax=[]  KbParamMin=[]  KbParamMax=[]  KtParamMin=[]  KtParamMax=[]  KbOutMin=[]  KbOutMax=[]  KtOutMin=[]  KtOutMax=[]  IntegratorOutMin=[]  IntegratorOutMax=[]  FilterOutMin=[]  FilterOutMax=[]  SumI1OutMin=[]  SumI1OutMax=[]  SumI2OutMin=[]  SumI2OutMax=[]  SumI3OutMin=[]  SumI3OutMax=[]  SumI4OutMin=[]  SumI4OutMax=[]  SumDOutMin=[]  SumDOutMax=[]  DifferentiatorOutMin=[]  DifferentiatorOutMax=[]  FilterDiffOutCoefMin=[]  FilterDiffOutCoefMax=[]  ReciprocalOutMin=[]  ReciprocalOutMax=[]  SumDenOutMin=[]  SumDenOutMax=[]  SumNumOutMin=[]  SumNumOutMax=[]  DivideOutMin=[]  DivideOutMax=[]  UdiffTsProdOutMin=[]  UdiffTsProdOutMax=[]  NTsProdOutMin=[]  NTsProdOutMax=[]  UintegralTsProdOutMin=[]  UintegralTsProdOutMax=[]  UngainTsProdOutMin=[]  UngainTsProdOutMax=[]  ClampingZeroOutDataTypeStr=Inherit: Inherit via back propagation  ClampingZeroOutMin=[]  ClampingZeroOutMax=[]  FilterDenConstantOutDataTypeStr=Inherit: Inherit via back propagation  FilterDenConstantOutMin=[]  FilterDenConstantOutMax=[]  PCopyOutDataTypeStr=Inherit: Inherit via back propagation  PCopyOutMin=[]  PCopyOutMax=[]  NCopyOutDataTypeStr=Inherit: Inherit via back propagation  NCopyOutMin=[]  NCopyOutMax=[]  IntegratorContinuousStateAttributes=''  IntegratorStateMustResolveToSignalObject=off  IntegratorRTWStateStorageClass=Auto  FilterContinuousStateAttributes=''  FilterStateMustResolveToSignalObject=off  FilterRTWStateStorageClass=Auto  ParallelPVariant=InternalParameters  IdealPVariant=Disabled  IVariant=InternalParameters  DVariant=Disabled  IntegratorVariant=Discrete  SatVariant=Disabled  AWVariant=Passthrough  PCopyVariant=Disabled  TRVariant=Disabled  FdbkBlocksVariant=Forward  IdealPFdbkVariant=Disabled  SatFdbkVariant=Disabled  DerivativeFilterVariant=Disabled  NVariant=Disabled  NCopyVariant=Disabled_SignalSpec  FilterICVariant=Disabled  IntegratorICVariant=InternalICs  ExternalResetVariant=ExternalReset  TRSumVariant=Passthrough  SumFdbkVariant=Disabled  SumVariant=Sum_PI  TsampFilterVariant=InternalTs  TsampNgainVariant=Passthrough  TsampIntegralVariant=Disabled_SignalSpec  ExternalSaturationOutDataTypeStr=Inherit: Same as second input  DerivativeSourceVariant=Disabled  PreIntVariant=InternalPreInt
  Sin : Trigonometry
  Sum3 : Sum  Inputs=-+|
  Sum4 : Sum  Inputs=-+|
  Sum6 : Sum  Inputs=|+-
  delta_theta : Outport
  delta_wt : Outport  Port=2
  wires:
  Delay/1 -> Sum3/1
  Sin/1 -> MATLAB Function/1(error)
  sync/1 -> MATLAB Function1/2(sync), MATLAB Function2/2(sync), Compare To Zero/1, Compare To Zero1/1
  [theta_gfm_2] -> Sum4/1
  Sum6/1 -> MATLAB Function/2(error_w)
  MATLAB Function2/1(y) -> delta_wt/1  "delta_wt"
  connect/1 -> MATLAB Function/3(reset)
  PID Controller/1 -> MATLAB Function2/1(u)  "delta_w"
  Sum3/1 -> PID Controller/1, [w_err]  "err_w"
  w_pcc/1 -> Sum3/2, Sum6/1
  Sum4/1 -> Sin/1, [theta_err]
  Compare To Zero1/1 -> PID Controller1/2
  MATLAB Function/1(y) -> PID Controller1/1
  PID Controller1/1 -> MATLAB Function1/1(u)  "delta_theta"
  Compare To Zero/1 -> PID Controller/2
  [w] -> Delay/1
  theta_pcc/1 -> Sum4/2
  MATLAB Function1/1(y) -> delta_theta/1  "delta_theta"
  [w] -> Delay1/1
  Delay1/1 -> Sum6/2

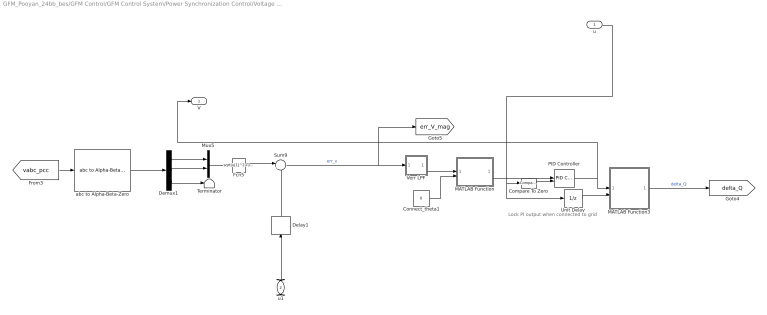
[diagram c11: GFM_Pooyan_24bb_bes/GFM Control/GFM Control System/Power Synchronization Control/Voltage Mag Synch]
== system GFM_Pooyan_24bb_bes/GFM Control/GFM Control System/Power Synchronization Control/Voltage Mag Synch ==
  note: Lock PI output when connected to grid
  u : Inport
  u1 : Inport  Port=2
  Compare To Zero : simulink/Logic and Bit Operations/Compare To Zero  relop===  OutDataTypeStr=boolean
  Connect_theta1 : Constant  Value=0
  Delay1 : Delay  DelayLength=1  InputProcessing=Columns as channels (frame based)
  Demux1 : Demux  Outputs=3
  Fcn5 : Fcn  Expr=sqrt(u[1]^2+u[2]^2)
  MATLAB Function : MATLAB Function  TreatAsAtomicUnit=on
  MATLAB Function3 : MATLAB Function  TreatAsAtomicUnit=on
  Mux5 : Mux  Inputs=2
  PID Controller : slpidlib/PID Controller  Controller=PID  Form=Parallel  TimeDomain=Discrete-time  UseExternalTs=off  SampleTime=-1  IntegratorMethod=Forward Euler  FilterMethod=Forward Euler  ControllerParametersSource=internal  P=0.23  I=20  UseKiTs=off  D=0  UseExternalDerivativeSource=off  N=100  UseFilter=on  TunerSelectOption=Transfer Function Based (PID Tuner App)  InitialConditionSource=internal  InitialConditionForIntegrator=0  InitialConditionForFilter=0  DifferentiatorICPrevScaledInput=0  ExternalReset=level  TrackingMode=off  Kt=1  LimitOutput=off  SatLimitsSource=internal  UpperSaturationLimit=inf  LowerSaturationLimit=-inf  LinearizeAsGain=on  AntiWindupMode=none  Kb=1  LimitIntegrator=off  UpperIntegratorSaturationLimit=inf  LowerIntegratorSaturationLimit=-inf  POutMin=[]  POutMax=[]  IOutMin=[]  IOutMax=[]  DOutMin=[]  DOutMax=[]  NOutMin=[]  NOutMax=[]  SumOutMin=[]  SumOutMax=[]  SaturationOutMin=[]  SaturationOutMax=[]  PParamMin=[]  PParamMax=[]  IParamMin=[]  IParamMax=[]  DParamMin=[]  DParamMax=[]  NParamMin=[]  NParamMax=[]  KbParamMin=[]  KbParamMax=[]  KtParamMin=[]  KtParamMax=[]  KbOutMin=[]  KbOutMax=[]  KtOutMin=[]  KtOutMax=[]  IntegratorOutMin=[]  IntegratorOutMax=[]  FilterOutMin=[]  FilterOutMax=[]  SumI1OutMin=[]  SumI1OutMax=[]  SumI2OutMin=[]  SumI2OutMax=[]  SumI3OutMin=[]  SumI3OutMax=[]  SumI4OutMin=[]  SumI4OutMax=[]  SumDOutMin=[]  SumDOutMax=[]  DifferentiatorOutMin=[]  DifferentiatorOutMax=[]  FilterDiffOutCoefMin=[]  FilterDiffOutCoefMax=[]  ReciprocalOutMin=[]  ReciprocalOutMax=[]  SumDenOutMin=[]  SumDenOutMax=[]  SumNumOutMin=[]  SumNumOutMax=[]  DivideOutMin=[]  DivideOutMax=[]  UdiffTsProdOutMin=[]  UdiffTsProdOutMax=[]  NTsProdOutMin=[]  NTsProdOutMax=[]  UintegralTsProdOutMin=[]  UintegralTsProdOutMax=[]  UngainTsProdOutMin=[]  UngainTsProdOutMax=[]  ClampingZeroOutDataTypeStr=Inherit: Inherit via back propagation  ClampingZeroOutMin=[]  ClampingZeroOutMax=[]  FilterDenConstantOutDataTypeStr=Inherit: Inherit via back propagation  FilterDenConstantOutMin=[]  FilterDenConstantOutMax=[]  PCopyOutDataTypeStr=Inherit: Inherit via back propagation  PCopyOutMin=[]  PCopyOutMax=[]  NCopyOutDataTypeStr=Inherit: Inherit via back propagation  NCopyOutMin=[]  NCopyOutMax=[]  IntegratorContinuousStateAttributes=''  IntegratorStateMustResolveToSignalObject=off  IntegratorRTWStateStorageClass=Auto  FilterContinuousStateAttributes=''  FilterStateMustResolveToSignalObject=off  FilterRTWStateStorageClass=Auto  ParallelPVariant=InternalParameters  IdealPVariant=Disabled  IVariant=InternalParameters  DVariant=InternalParameters  IntegratorVariant=Discrete  SatVariant=Disabled  AWVariant=Passthrough  PCopyVariant=Disabled  TRVariant=Disabled  FdbkBlocksVariant=Forward  IdealPFdbkVariant=Disabled  SatFdbkVariant=Disabled  DerivativeFilterVariant=ForwardEulerFilter  NVariant=InternalParameters  NCopyVariant=Disabled  FilterICVariant=InternalICsFilter  IntegratorICVariant=InternalICs  ExternalResetVariant=ExternalReset  TRSumVariant=Passthrough  SumFdbkVariant=Disabled  SumVariant=Sum_PID  TsampFilterVariant=InternalTs  TsampNgainVariant=Passthrough  TsampIntegralVariant=Disabled_SignalSpec  ExternalSaturationOutDataTypeStr=Inherit: Same as second input  DerivativeSourceVariant=ErrorSignal  PreIntVariant=InternalPreInt
  Sum9 : Sum  Inputs=|+-
  Terminator : Terminator
  Unit Delay : UnitDelay  SampleTime=-1  HasFrameUpgradeWarning=on
  Verr LPF : Subsystem  mask{fc=10}
      mask prompts: fc "Cut-off frequency [Hz]"
      mask help: 1st-order IIR LPF
  abc to Alpha-Beta-Zero : spsabctoAlphaBetaZeroLib/abc to Alpha-Beta-Zero
  V : Outport
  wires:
  Unit Delay/1 -> MATLAB Function3/2(sync)
  [vabc_pcc] -> abc to Alpha-Beta-Zero/1
  u/1 -> Compare To Zero/1, Unit Delay/1
  MATLAB Function3/1(y) -> [delta_Q]  "delta_Q"
  PID Controller/1 -> V/1, MATLAB Function3/1(u)
  abc to Alpha-Beta-Zero/1 -> Demux1/1
  Demux1/1 -> Mux5/1
  Demux1/2 -> Mux5/2
  Demux1/3 -> Terminator/1
  MATLAB Function/1(y) -> PID Controller/1
  u1/1 -> Delay1/1
  Connect_theta1/1 -> MATLAB Function/2(reset)
  Sum9/1 -> Verr LPF/1(In), [err_V_mag]  "err_v"
  Delay1/1 -> Sum9/2
  Verr LPF/1(Out) -> MATLAB Function/1(error)
  Fcn5/1 -> Sum9/1
  Mux5/1 -> Fcn5/1
  Compare To Zero/1 -> PID Controller/2

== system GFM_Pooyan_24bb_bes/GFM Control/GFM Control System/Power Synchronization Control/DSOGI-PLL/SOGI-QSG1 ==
  Va : Inport
  f : Inport  Port=2
  2*pi : Gain  Gain=2*pi
  Divide1 : Product  Inputs=**
  Divide2 : Product  Inputs=**
  Integrator : Integrator
  Integrator1 : Integrator
  K : Gain  Gain=0.8
  Sum1 : Sum  Inputs=|+-
  Sum2 : Sum  Inputs=-+|
  vad : Outport  VectorParamsAs1DForOutWhenUnconnected=off
  vaq : Outport  Port=2  VectorParamsAs1DForOutWhenUnconnected=off
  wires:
  2*pi/1 -> Divide1/2, Divide2/2
  Va/1 -> Sum2/2
  Integrator1/1 -> vaq/1, Sum1/2
  Divide2/1 -> Integrator1/1
  Integrator/1 -> vad/1, Divide2/1, Sum2/1
  Sum2/1 -> K/1
  K/1 -> Sum1/1
  Sum1/1 -> Divide1/1
  Divide1/1 -> Integrator/1
  f/1 -> 2*pi/1

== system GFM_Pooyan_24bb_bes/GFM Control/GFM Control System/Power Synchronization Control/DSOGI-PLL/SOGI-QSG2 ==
  f : Inport
  Vb : Inport  Port=2
  2*pi : Gain  Gain=2*pi
  Divide1 : Product  Inputs=**
  Divide2 : Product  Inputs=**
  Integrator : Integrator
  Integrator1 : Integrator
  K : Gain  Gain=0.8
  Sum1 : Sum  Inputs=|+-
  Sum2 : Sum  Inputs=-+|
  vbd : Outport  VectorParamsAs1DForOutWhenUnconnected=off
  vbq : Outport  Port=2  VectorParamsAs1DForOutWhenUnconnected=off
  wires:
  Divide1/1 -> Integrator/1
  Sum1/1 -> Divide1/1
  K/1 -> Sum1/1
  Sum2/1 -> K/1
  Integrator/1 -> Sum2/1, Divide2/1, vbd/1
  Divide2/1 -> Integrator1/1
  Integrator1/1 -> Sum1/2, vbq/1
  Vb/1 -> Sum2/2
  2*pi/1 -> Divide2/2, Divide1/2
  f/1 -> 2*pi/1
